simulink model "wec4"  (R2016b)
settings: Solver=ode4  StartTime=0  StopTime=1000  FixedStep=0.005  MaxStep=0.005  RelTol=1e-3  EnableMultiTasking=on
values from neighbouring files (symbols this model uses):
  arAdaptiveLawData = 1/2*zModelSimple.zModelPto.arFreq.*     zModelSimple.zModelPto.arMagnitude./     cos(zModelSimple.zModelPto.arPhase*pi/180+pi/2)    [IMPACT_Control.m]
  arAdaptiveLawDataX = 1/2*zModelSimpleX.zModelPto.arFreq.*         zModelSimpleX.zModelPto.arMagnitude./         cos(zModelSimpleX.zModelPto.arPhase*pi/180+pi/2)    [IMPACT_Control.m]
  arControllerRampGain = [0,0,1,1]    [IMPACT_Control.m]
  arControllerRampTime = [0 rStartRampTime rStartRampTime+rRampTimeLength 8000]    [IMPACT_Control.m]
  arEkfInitialisation = zeros(1,11)    [IMPACT_Control.m]
  arEkfInitialisationX = zeros(1,11)    [IMPACT_Control.m]
  arFrequency = zModelSimple.zModelPto.arFreq    [IMPACT_Control.m]
  arFrequencyRange = zModelSimple.zModelPto.arFreq    [IMPACT_Control.m]
  arFrequencyX = zModelSimpleX.zModelPto.arFreq    [IMPACT_Control.m]
  arImpedance = 1./zModelSimple.zModelPto.arMagnitude./zModelSimple.zModelPto.arFreq    [IMPACT_Control.m]
  arImpedanceX = 1./zModelSimpleX.zModelPto.arMagnitude./zModelSimpleX.zModelPto.arFreq    [IMPACT_Control.m]
  CentralPTOPreload = -1.6113e+07    (= -16113000)    [wecSimInputFile.m]
  F1 = [4.243 2.375 -12.243]    [wecSimInputFile.m]
  F2 = [4.243 -2.375 -12.243]    [wecSimInputFile.m]
  F3 = [-4.243 -2.375 -12.243]    [wecSimInputFile.m]
  F4 = [-4.243 2.375 -12.243]    [wecSimInputFile.m]
  FC = [0 0 -14]    [wecSimInputFile.m]
  iAdaptiveDamping = 0    [wec4IMPACT_Project.m]    (also in IMPACT_Control.m = handles.iAdaptiveDamping; wec1_IMPACT_Project.m; wec2_IMPACT_Project.m; wec3_IMPACT_Project.m)
  iControlType = 2    [wec4IMPACT_Project.m]    (also in IMPACT_Control.m = handles.iControlType; wec1_IMPACT_Project.m = 1; wec2_IMPACT_Project.m = 1; wec3_IMPACT_Project.m = 1)
  iPtoPositionConstraint = 1    [wec4IMPACT_Project.m]    (also in IMPACT_Control.m = handles.iPtoPositionConstraint; wec1_IMPACT_Project.m = 0; wec2_IMPACT_Project.m; wec3_IMPACT_Project.m)
  iSensorNoise = 0    [IMPACT_Control.m]
  m = m+1    (= 2)    [checkParamFile.m]
  PTOrotation = atan((T1(2)-F1(2))/(T1(1)-F1(1)))    [wecSimInputFile.m]
  rCogFloater = -8    [wec4_IMPACT_Model.m]    (also in paramInitial.m = get( handles.edit_rCogFloater, 'String' ); wec1_IMPACT_Model.m = -18; wec2_IMPACT_Model.m = -8.5; wec3_IMPACT_Model.m = -0.7)
  rCogSpar = -36.6    [wec4_IMPACT_Model.m]    (also in paramInitial.m = get( handles.edit_rCogSpar, 'String' ); wec3_IMPACT_Model.m = -21.3; wec3_IMPACT_Model2.m = -21.3)
  rDisplacementLimit = 10.000000    (= 10)    [wec4IMPACT_Project.m]    (also in IMPACT_Control.m = getValue(handles.edit_displacementLimit); wec1_IMPACT_Project.m; wec2_IMPACT_Project.m; wec3_IMPACT_Project.m = 3)
  rDisplacementLimitX = 10.000000    (= 10)    [wec4IMPACT_Project.m]    (also in IMPACT_Control.m = getValue(handles.edit_displacementLimitX); wec1_IMPACT_Project.m = 0; wec2_IMPACT_Project.m; wec3_IMPACT_Project.m = 0)
  rGainForAntiWIndUp = tfControllerDiscrete.rGain    [IMPACT_Control.m]
  rGainForAntiWIndUpX = tfControllerXDiscrete.rGain    [IMPACT_Control.m]
  rMaxForcePto = 300000000.000000    (= 300000000)    [wec4IMPACT_Project.m]    (also in IMPACT_Control.m = getValue(handles.edit_maxForcePto); wec1_IMPACT_Project.m = 1e+15; wec2_IMPACT_Project.m = 1e+15; wec3_IMPACT_Project.m = 1000000000)
  rMinForcePto = -300000000.000000    (= -300000000)    [wec4IMPACT_Project.m]    (also in IMPACT_Control.m = getValue(handles.edit_minForcePto); wec1_IMPACT_Project.m = -1e+15; wec2_IMPACT_Project.m = -1e+15; wec3_IMPACT_Project.m = -1000000000)
  rMooringX = 20000    [wec4_IMPACT_Model.m]    (also in paramInitial.m = get( handles.edit_rMooringX, 'String' ); wec3_IMPACT_Model.m = 10000; wec3_IMPACT_Model2.m = 10000)
  rMooringZ = 10000    [wec4_IMPACT_Model.m]    (also in paramInitial.m = get( handles.edit_rMooringZ, 'String' ); wec3_IMPACT_Model.m = 0; wec3_IMPACT_Model2.m = 0)
  rOutputSampleTime = 0.010000    (= 0.01)    [wec4IMPACT_Project.m]    (also in IMPACT_Control.m = getValue(handles.edit_outputSampleTime); wec1_IMPACT_Project.m; wec2_IMPACT_Project.m; wec3_IMPACT_Project.m)
  rPassiveDampingGain = -604830.000000    (= -604830)    [wec4IMPACT_Project.m]    (also in IMPACT_Control.m = getValue(handles.edit_gainPLD); wec1_IMPACT_Project.m = -214018.1537; wec2_IMPACT_Project.m = -1948070; wec3_IMPACT_Project.m = -519390)
  rPassiveDampingGainX = -278660.000000    (= -278660)    [wec4IMPACT_Project.m]    (also in IMPACT_Control.m = getValue(handles.edit_gainPLDX); wec1_IMPACT_Project.m = 0; wec2_IMPACT_Project.m = 0; wec3_IMPACT_Project.m = 0)
  rTetherPretension = 1.6113e+07    (= 16113000)    [wec4_IMPACT_Model.m]    (also in paramInitial.m = get( handles.edit_rTetherPretension, 'String' ); wec3_IMPACT_Model.m = 0; wec3_IMPACT_Model2.m = 0)
  rTetherSpring = 500000    [wec4_IMPACT_Model.m]    (also in paramInitial.m = get( handles.edit_rTetherSpring, 'String' ); wec3_IMPACT_Model.m = 0; wec3_IMPACT_Model2.m = 0)
  rUpperFrequencyLimit = EKFFloater.upperFreq    [IMPACT_Control.m]
  rXf = 4.243    [wec4AdditionalParams.m]
  rXs = 16.075    [wec4AdditionalParams.m]
  rYf = 2.375    [wec4AdditionalParams.m]
  rYs = 16.075    [wec4AdditionalParams.m]
  rZf = 4.243    [wec4AdditionalParams.m]
  rZs = 2.4350    (= 2.435)    [wec4AdditionalParams.m]
  rZTetherF = 6    [wec4AdditionalParams.m]
  rZTetherS = 2.4350    (= 2.435)    [wec4AdditionalParams.m]
  s = tf('s')    [wec4_IMPACT_Model.m]    (also in IMPACT_Control.m; wec1_IMPACT_Model.m; wec2_IMPACT_Model.m; wec3_IMPACT_Model.m)
  SidePTO1Preload = PreloadPTOCorner    (= 0)    [wecSimInputFile.m]
  SidePTO2Preload = PreloadPTOCorner    (= 0)    [wecSimInputFile.m]
  SidePTO3Preload = PreloadPTOCorner    (= 0)    [wecSimInputFile.m]
  SidePTO4Preload = PreloadPTOCorner    (= 0)    [wecSimInputFile.m]
  simu = simulationClass()    [wecSimInputFile.m]
  T1 = [16.075 16.075 -34.165]    [wecSimInputFile.m]
  T2 = [16.075 -16.075 -34.165]    [wecSimInputFile.m]
  T3 = [-16.075 -16.075 -34.165]    [wecSimInputFile.m]
  T4 = [-16.075 16.075 -34.165]    [wecSimInputFile.m]
  TC = [0 0 -34.165]    [wecSimInputFile.m]
  waves = waveClass('irregular')    [wecSimInputFile.m]
  Z = magPhaseToComplex(zModelTf)    [IMPACT_Control.m]
undefined symbols (not defined in the file or in its folder): arControllerDiscreteDen, arControllerDiscreteNum, arControllerDiscreteXDen, arControllerDiscreteXNum, arExcForceFloaterDen, arExcForceFloaterNum, arExcForceFloaterXDen, arExcForceFloaterXNum, arExcForceSparDen, arExcForceSparNum, arExcForceSparXDen, arExcForceSparXNum, arFexcFloaterDen, arFexcFloaterNum, arFexcFloaterXDen, arFexcFloaterXNum, arFexcSparDen, arFexcSparNum, arFexcSparXDen, arFexcSparXNum, Body, body, constraint, CTTime, deg, Elements, geometry, IRKB, kg, lenJ, mooring, N, pto, rAccelerationGainFloater, rAccelerationGainFloaterX, rAccelerationGainSpar, rAccelerationGainSparX, rad, rBuoyancyGainFloater, rBuoyancyGainFloaterX, rBuoyancyGainSpar, rBuoyancyGainSparX, rDampingGainFloater, rDampingGainFloaterX, rDampingGainSpar, rDampingGainSparX, Rigid, rMaxFocePto, wec4_float, wec4_reactor, WECSim_Lib, X, Y
libraries: nesl_utility x380, sm_lib x170, vrlib x91, simulink x12, WECSim_Lib x4
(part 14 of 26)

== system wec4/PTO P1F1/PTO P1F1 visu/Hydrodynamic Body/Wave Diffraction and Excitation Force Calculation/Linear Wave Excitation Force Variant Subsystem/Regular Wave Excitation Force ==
  note: Calculates the wave force, F_wave, for the case of Regular Waves. F_wave = A * cos(w * t) * Re{Fext} - A * sin(w * t) * Im{Fext}
  In1 : Inport
  Add : Sum
  Add1 : Sum  Inputs=+-
  Constant : Constant  Value=pi/2
  Excitation Imaginary Part : Constant  Value=body.hydroForce.fExt.im(1,:)  VectorParams1D=off
  Excitation Real Part : Constant  Value=body.hydroForce.fExt.re(1,:)  VectorParams1D=off
  Product : Product
  Product1 : Product  Inputs=3
  Product2 : Product  Inputs=3
  Sine Wave Function : Sin  TimeSource=Use external signal  SampleTime=0
  Sine Wave Function1 : Sin  TimeSource=Use external signal  SampleTime=0
  Wave Amplitude : Constant  Value=waves.A(1,:)
  Wave Frequency : Constant  Value=waves.w(1,:)
  Out1 : Outport
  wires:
  Constant/1 -> Add/2
  Add/1 -> Sine Wave Function1/1
  Wave Amplitude/1 -> Product1/1, Product2/1  "A"
  Add1/1 -> Out1/1
  Product2/1 -> Add1/2
  Product1/1 -> Add1/1
  Excitation Real Part/1 -> Product1/2  "Re{Fext}"
  Excitation Imaginary Part/1 -> Product2/3  "Im{Fext}"
  Sine Wave Function/1 -> Product2/2  "sin(wt)"
  Sine Wave Function1/1 -> Product1/3  "cos(w*t)"
  Product/1 -> Add/1, Sine Wave Function/1
  Wave Frequency/1 -> Product/2  "w"
  In1/1 -> Product/1  "t"

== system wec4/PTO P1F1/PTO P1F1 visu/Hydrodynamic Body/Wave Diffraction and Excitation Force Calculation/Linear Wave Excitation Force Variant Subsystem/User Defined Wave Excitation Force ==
  note: Calculates the wave force, F_wave, for the case of User Defined Waves. F_wave = convolution calculation [1x6]
  InputWaveForceTimeHistory : FromWorkspace  VariableName=[waves.waveAmpTime(:,1),body.hydroForce.userDefinedFe]  SampleTime=0
  Out1 : Outport
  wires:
  InputWaveForceTimeHistory/1 -> Out1/1

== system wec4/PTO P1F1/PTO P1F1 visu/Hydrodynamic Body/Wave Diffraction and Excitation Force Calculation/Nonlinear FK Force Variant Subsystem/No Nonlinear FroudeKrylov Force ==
  Constant : Constant  Value=[0 0 0 0 0 0]
  Out1 : Outport
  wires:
  Constant/1 -> Out1/1

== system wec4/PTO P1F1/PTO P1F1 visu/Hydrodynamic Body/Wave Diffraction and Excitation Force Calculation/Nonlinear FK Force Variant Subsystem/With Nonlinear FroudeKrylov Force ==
  In1 : Inport
  In2 : Inport  Port=2
  In3 : Inport  Port=3
  Add : Sum  Inputs=+-
  Center of Gravity : Constant  Value=body.hydroData.properties.cg
  Center of Gravity1 : Constant  Value=body.hydroData.properties.cg
  Constant : Constant  Value=[0 0 0]
  Deep Water Flag : Constant  Value=waves.deepWaterWave
  Diffraction and Excitation Forces : MATLAB Function  TreatAsAtomicUnit=on
  Frequency Spacing : Constant  Value=waves.dw
  Gravity : Constant  Value=simu.g
  Mux : Mux  Inputs=2
  STL Areas : Constant  Value=body.bodyGeometry.area
  STL Centers : Constant  Value=body.bodyGeometry.center
  STL Normal Vectors : Constant  Value=body.bodyGeometry.norm
  To Workspace : ToWorkspace  VariableName=body4_wavenonlinearpressure_out  SaveFormat=Structure With Time  SampleTime=-1
  To Workspace1 : ToWorkspace  VariableName=body4_wavelinearpressure_out  SaveFormat=Structure With Time  SampleTime=-1
  Water Density : Constant  Value=simu.rho
  Water Depth : Constant  Value=waves.waterDepth
  Wave Amplitude : Constant  Value=waves.A
  Wave Frequency : Constant  Value=waves.w
  Wave Number : Constant  Value=waves.k
  Wave Random Phase : Constant  Value=waves.phase
  Wave Type Number : Constant  Value=waves.typeNum
  Out1 : Outport
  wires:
  STL Areas/1 -> Diffraction and Excitation Forces/5(area)
  Diffraction and Excitation Forces/2(wp) -> To Workspace/1
  Diffraction and Excitation Forces/3(wpMeanFS) -> To Workspace1/1
  In2/1 -> Add/1
  Constant/1 -> Mux/2
  Center of Gravity/1 -> Mux/1  "cg"
  Mux/1 -> Add/2
  Add/1 -> Diffraction and Excitation Forces/1(x)  "x_cg"
  Deep Water Flag/1 -> Diffraction and Excitation Forces/13(deepWaterWave)
  Wave Random Phase/1 -> Diffraction and Excitation Forces/17(phaseRand)
  Water Depth/1 -> Diffraction and Excitation Forces/12(wDepth)
  Wave Number/1 -> Diffraction and Excitation Forces/14(k)
  Wave Type Number/1 -> Diffraction and Excitation Forces/15(typeNum)
  Frequency Spacing/1 -> Diffraction and Excitation Forces/11(dw)
  Wave Frequency/1 -> Diffraction and Excitation Forces/10(w)
  Wave Amplitude/1 -> Diffraction and Excitation Forces/9(AH)
  In1/1 -> Diffraction and Excitation Forces/16(t)
  In3/1 -> Diffraction and Excitation Forces/2(elv)
  STL Centers/1 -> Diffraction and Excitation Forces/3(center)
  STL Normal Vectors/1 -> Diffraction and Excitation Forces/4(tnorm)
  Water Density/1 -> Diffraction and Excitation Forces/6(rho)
  Gravity/1 -> Diffraction and Excitation Forces/7(g)
  Diffraction and Excitation Forces/1(f) -> Out1/1
  Center of Gravity1/1 -> Diffraction and Excitation Forces/8(cg)

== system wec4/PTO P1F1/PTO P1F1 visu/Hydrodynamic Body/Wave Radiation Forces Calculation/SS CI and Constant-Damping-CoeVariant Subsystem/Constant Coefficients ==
  In1 : Inport
  Product : Product  Multiplication=Matrix(*)
  Radiation Damping Matrix : Constant  Value=body.hydroForce.fDamping
  Out1 : Outport
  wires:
  In1/1 -> Product/2
  Product/1 -> Out1/1  "F_Single Frequency"
  Radiation Damping Matrix/1 -> Product/1

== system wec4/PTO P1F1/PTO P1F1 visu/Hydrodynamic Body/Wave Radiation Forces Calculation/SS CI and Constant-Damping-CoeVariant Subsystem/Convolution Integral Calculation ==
  In1 : Inport
  MATLAB Function : MATLAB Function  TreatAsAtomicUnit=on  SystemSampleTime=simu.CTTime(2) - simu.CTTime(1)
  Rate Transition : RateTransition
  Reshape : Reshape
  Out1 : Outport
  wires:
  Rate Transition/1 -> Reshape/1
  MATLAB Function/1(F_FM) -> Rate Transition/1
  Reshape/1 -> Out1/1
  In1/1 -> MATLAB Function/1(v)

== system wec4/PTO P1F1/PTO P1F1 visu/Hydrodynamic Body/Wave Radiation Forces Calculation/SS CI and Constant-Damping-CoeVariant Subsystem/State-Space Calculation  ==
  In1 : Inport
  State-Space : StateSpace  A=body.hydroForce.ssRadf.A  B=body.hydroForce.ssRadf.B  C=body.hydroForce.ssRadf.C  D=body.hydroForce.ssRadf.D  X0=0
  Out1 : Outport
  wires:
  State-Space/1 -> Out1/1
  In1/1 -> State-Space/1  "x"

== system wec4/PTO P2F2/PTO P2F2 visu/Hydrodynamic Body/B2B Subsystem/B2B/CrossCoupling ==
  note: CrossCoupling block is updated by its mask initialization, which is only called on when a simulation is run. 'From' blocks are automatically created and connected based on the number of bodies in the simulation.
  Mux1 : Mux  Inputs=2
  Mux2 : Mux  Inputs=2
  vel : Outport
  acc : Outport  Port=2
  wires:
  [acc2] -> Mux2/2
  Mux2/1 -> acc/1
  [acc1] -> Mux2/1
  [vel2] -> Mux1/2
  Mux1/1 -> vel/1
  [vel1] -> Mux1/1

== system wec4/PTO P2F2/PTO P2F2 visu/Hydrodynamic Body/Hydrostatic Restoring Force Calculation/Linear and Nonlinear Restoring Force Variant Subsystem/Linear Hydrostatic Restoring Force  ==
  In1 : Inport
  Add1 : Sum  Inputs=+-
  Add2 : Sum  Inputs=+++
  Add3 : Sum  Inputs=+-
  Assignment (Add Net Bouyancy Force to Z-Direction) : Assignment  IndexOptions=Index vector (dialog)  Indices=3  OutputSizes=1
  Assignment (Add Net Bouyancy Force to Z-Direction)1 : Assignment  IndexOptions=Index vector (dialog)  Indices=3  OutputSizes=1
  Assignment (Add Net Bouyancy Force to Z-Direction)2 : Assignment  IndexOptions=Index vector (dialog)  Indices=4:6  OutputSizes=1
  Body Mass : Constant  Value=body.hydroForce.storage.mass
  Center of Gravity : Constant  Value=body.cg
  Center of Gravity1 : Constant  Value=body.cb
  Constant1 : Constant  Value=[0 0 0 0 0 0]
  Constant2 : Constant  Value=[0 0 0]
  Cross Product : vrlib/Utilities/Cross Product
  Gravity : Constant  Value=simu.g
  Linear Restioring Coefficient Matrix : Constant  Value=body.hydroForce.linearHydroRestCoef
  Product : Product
  Product1 : Product  Inputs=3
  Product2 : Product  Multiplication=Matrix(*)
  Volume : Constant  Value=body.dispVol
  Water Density : Constant  Value=simu.rho
  Out1 : Outport
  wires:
  Assignment (Add Net Bouyancy Force to Z-Direction)2/1 -> Add2/3
  Constant1/1 -> Assignment (Add Net Bouyancy Force to Z-Direction)/1, Assignment (Add Net Bouyancy Force to Z-Direction)2/1
  Cross Product/1 -> Assignment (Add Net Bouyancy Force to Z-Direction)2/2
  Assignment (Add Net Bouyancy Force to Z-Direction)1/1 -> Cross Product/1
  Constant2/1 -> Assignment (Add Net Bouyancy Force to Z-Direction)1/1
  Add3/1 -> Cross Product/2
  Center of Gravity/1 -> Add3/2  "cg"
  Center of Gravity1/1 -> Add3/1  "x"
  Linear Restioring Coefficient Matrix/1 -> Product2/1  "K"
  Product2/1 -> Add2/2  "Linear Restoring Force"
  Add1/1 -> Assignment (Add Net Bouyancy Force to Z-Direction)/2
  Product1/1 -> Assignment (Add Net Bouyancy Force to Z-Direction)1/2, Add1/2  "F_Buoyancy"
  Product/1 -> Add1/1  "F_Gravity"
  Water Density/1 -> Product1/1  "rho"
  Gravity/1 -> Product/1, Product1/2  "g"
  Volume/1 -> Product1/3  "Vol"
  Add2/1 -> Out1/1  "F_Restoring"
  Assignment (Add Net Bouyancy Force to Z-Direction)/1 -> Add2/1  "Net Buoyancy Force"
  Body Mass/1 -> Product/2  "m"
  In1/1 -> Product2/2  "x"

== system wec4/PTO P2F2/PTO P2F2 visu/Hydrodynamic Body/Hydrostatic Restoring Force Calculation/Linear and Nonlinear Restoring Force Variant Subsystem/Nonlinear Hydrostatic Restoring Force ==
  In1 : Inport
  In2 : Inport  Port=2
  Body Mass2 : Constant  Value=body.hydroForce.storage.mass
  Center of Gravity : Constant  Value=body.cg
  Gravity2 : Constant  Value=simu.g
  Rate Transition : RateTransition
  Rate Transition1 : RateTransition
  Restoring Forces : MATLAB Function  TreatAsAtomicUnit=on  SystemSampleTime=simu.dtNL
  STL areas : Constant  Value=body.bodyGeometry.area
  STL centers : Constant  Value=body.bodyGeometry.center
  STL normal vectors : Constant  Value=body.bodyGeometry.norm
  To Workspace1 : ToWorkspace  VariableName=body5_hspressure_out  SaveFormat=Structure With Time  SampleTime=-1
  Water Density1 : Constant  Value=simu.rho
  Out1 : Outport
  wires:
  Rate Transition/1 -> Out1/1
  Restoring Forces/1(f) -> Rate Transition/1
  Rate Transition1/1 -> To Workspace1/1
  Restoring Forces/2(p) -> Rate Transition1/1
  Body Mass2/1 -> Restoring Forces/9(mass)
  STL areas/1 -> Restoring Forces/5(area)
  In2/1 -> Restoring Forces/2(elv)
  STL centers/1 -> Restoring Forces/3(center)
  STL normal vectors/1 -> Restoring Forces/4(tnorm)
  Water Density1/1 -> Restoring Forces/6(rho)
  Gravity2/1 -> Restoring Forces/7(g)  "g"
  Center of Gravity/1 -> Restoring Forces/8(cg)
  In1/1 -> Restoring Forces/1(x)

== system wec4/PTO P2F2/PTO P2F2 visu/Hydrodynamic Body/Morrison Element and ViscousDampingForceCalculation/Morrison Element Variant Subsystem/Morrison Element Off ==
  Constant : Constant  Value=[0 0 0 0 0 0]
  morison_force : Outport
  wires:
  Constant/1 -> morison_force/1

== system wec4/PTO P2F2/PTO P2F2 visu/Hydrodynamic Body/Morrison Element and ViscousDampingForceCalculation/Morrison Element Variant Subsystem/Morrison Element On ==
  note: 1) Add Subsystem or Model blocks as valid variant choices. 2) You cannot connect blocks at this level. At simulation, connectivity is automatically determined, based on the active variant and port name matching.
  displacement : Inport
  velocity : Inport  Port=2
  acceleration : Inport  Port=3
  time : Inport  Port=4
  Irregular Wave Morison Force : Subsystem  TreatAsAtomicUnit=on  SystemSampleTime=simu.dtME  VariantControl=sv_irregularWaves
  No Wave Morison Force : Subsystem  VariantControl=sv_noWave
  Regular Wave Morison Force : Subsystem  TreatAsAtomicUnit=on  SystemSampleTime=simu.dtME  VariantControl=sv_regularWaves
  morison_force : Outport

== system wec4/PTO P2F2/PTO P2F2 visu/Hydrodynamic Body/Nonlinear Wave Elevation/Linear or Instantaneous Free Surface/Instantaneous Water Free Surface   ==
  In1 : Inport
  In2 : Inport  Port=2
  Center of Gravity : Constant  Value=body.cg
  Frequency Spacing : Constant  Value=waves.dw
  Instantaneous FS : MATLAB Function  TreatAsAtomicUnit=on
  Ramp Time : Constant  Value=simu.rampTime
  STL Centers : Constant  Value=body.bodyGeometry.center
  Wave Amplitude : Constant  Value=waves.A
  Wave Direction : Constant  Value=waves.waveDir
  Wave Frequency : Constant  Value=waves.w
  Wave Number : Constant  Value=waves.k
  Wave Random Phase : Constant  Value=waves.phase
  Wave Type Number : Constant  Value=waves.typeNum
  Out1 : Outport
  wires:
  Wave Amplitude/1 -> Instantaneous FS/4(AH)
  Wave Direction/1 -> Instantaneous FS/12(waveDir)
  In1/1 -> Instantaneous FS/1(x)
  In2/1 -> Instantaneous FS/9(t)
  Frequency Spacing/1 -> Instantaneous FS/6(dw)
  Wave Random Phase/1 -> Instantaneous FS/11(phaseRand)
  Ramp Time/1 -> Instantaneous FS/10(rampT)
  Wave Type Number/1 -> Instantaneous FS/8(typeNum)
  Wave Frequency/1 -> Instantaneous FS/5(w)
  Wave Number/1 -> Instantaneous FS/7(k)
  Center of Gravity/1 -> Instantaneous FS/3(cg)
  STL Centers/1 -> Instantaneous FS/2(center)
  Instantaneous FS/1(f) -> Out1/1

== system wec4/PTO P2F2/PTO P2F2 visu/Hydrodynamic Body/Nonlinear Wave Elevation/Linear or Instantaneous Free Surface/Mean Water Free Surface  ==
  zero : Constant  Value=0
  Out1 : Outport
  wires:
  zero/1 -> Out1/1

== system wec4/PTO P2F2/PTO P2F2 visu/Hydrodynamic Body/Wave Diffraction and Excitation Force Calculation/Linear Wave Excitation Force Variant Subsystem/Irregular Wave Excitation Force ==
  note: Calculates the wave force, F_wave, for the case of Irregular Waves. F_wave = sum( F_wave(i)) where i = each frequency bin.
  In1 : Inport
  Frequency Spacing Delta Omega : Constant  Value=waves.dw  VectorParams1D=off
  Imaginary Part of Wave Excitation : Constant  Value=body.hydroForce.fExt.im  VectorParams1D=off
  MATLAB Function : MATLAB Function  TreatAsAtomicUnit=on
  Random Phase : Constant  Value=waves.phase  VectorParams1D=off
  Real Part of Wave Excitation : Constant  Value=body.hydroForce.fExt.re  VectorParams1D=off
  Wave Frequency : Constant  Value=waves.w  VectorParams1D=off
  Wave Spectrum : Constant  Value=waves.A  VectorParams1D=off
  Out1 : Outport
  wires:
  Frequency Spacing Delta Omega/1 -> MATLAB Function/6(dw)
  In1/1 -> MATLAB Function/7(time)
  Wave Spectrum/1 -> MATLAB Function/1(A)
  Real Part of Wave Excitation/1 -> MATLAB Function/3(fExtRE)
  Imaginary Part of Wave Excitation/1 -> MATLAB Function/4(fExtIM)
  Wave Frequency/1 -> MATLAB Function/2(w)
  MATLAB Function/1(Fext) -> Out1/1
  Random Phase/1 -> MATLAB Function/5(phaseRand)

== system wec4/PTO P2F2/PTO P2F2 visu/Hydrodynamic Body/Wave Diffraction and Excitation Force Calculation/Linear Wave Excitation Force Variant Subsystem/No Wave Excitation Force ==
  Constant : Constant  Value=[0 0 0 0 0 0]
  Out1 : Outport
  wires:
  Constant/1 -> Out1/1

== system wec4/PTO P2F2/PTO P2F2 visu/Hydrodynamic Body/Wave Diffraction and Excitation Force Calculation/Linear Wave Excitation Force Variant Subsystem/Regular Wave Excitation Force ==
  note: Calculates the wave force, F_wave, for the case of Regular Waves. F_wave = A * cos(w * t) * Re{Fext} - A * sin(w * t) * Im{Fext}
  In1 : Inport
  Add : Sum
  Add1 : Sum  Inputs=+-
  Constant : Constant  Value=pi/2
  Excitation Imaginary Part : Constant  Value=body.hydroForce.fExt.im(1,:)  VectorParams1D=off
  Excitation Real Part : Constant  Value=body.hydroForce.fExt.re(1,:)  VectorParams1D=off
  Product : Product
  Product1 : Product  Inputs=3
  Product2 : Product  Inputs=3
  Sine Wave Function : Sin  TimeSource=Use external signal  SampleTime=0
  Sine Wave Function1 : Sin  TimeSource=Use external signal  SampleTime=0
  Wave Amplitude : Constant  Value=waves.A(1,:)
  Wave Frequency : Constant  Value=waves.w(1,:)
  Out1 : Outport
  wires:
  Constant/1 -> Add/2
  Add/1 -> Sine Wave Function1/1
  Wave Amplitude/1 -> Product1/1, Product2/1  "A"
  Add1/1 -> Out1/1
  Product2/1 -> Add1/2
  Product1/1 -> Add1/1
  Excitation Real Part/1 -> Product1/2  "Re{Fext}"
  Excitation Imaginary Part/1 -> Product2/3  "Im{Fext}"
  Sine Wave Function/1 -> Product2/2  "sin(wt)"
  Sine Wave Function1/1 -> Product1/3  "cos(w*t)"
  Product/1 -> Add/1, Sine Wave Function/1
  Wave Frequency/1 -> Product/2  "w"
  In1/1 -> Product/1  "t"

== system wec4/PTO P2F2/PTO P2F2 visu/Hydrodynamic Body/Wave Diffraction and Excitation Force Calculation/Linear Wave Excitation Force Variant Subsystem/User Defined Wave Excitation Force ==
  note: Calculates the wave force, F_wave, for the case of User Defined Waves. F_wave = convolution calculation [1x6]
  InputWaveForceTimeHistory : FromWorkspace  VariableName=[waves.waveAmpTime(:,1),body.hydroForce.userDefinedFe]  SampleTime=0
  Out1 : Outport
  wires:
  InputWaveForceTimeHistory/1 -> Out1/1

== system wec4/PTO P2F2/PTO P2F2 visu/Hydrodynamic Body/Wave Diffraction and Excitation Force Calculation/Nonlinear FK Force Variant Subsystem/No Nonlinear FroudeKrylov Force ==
  Constant : Constant  Value=[0 0 0 0 0 0]
  Out1 : Outport
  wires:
  Constant/1 -> Out1/1

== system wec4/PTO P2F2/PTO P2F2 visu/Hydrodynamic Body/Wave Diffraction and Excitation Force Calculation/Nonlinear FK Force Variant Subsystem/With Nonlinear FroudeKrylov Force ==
  In1 : Inport
  In2 : Inport  Port=2
  In3 : Inport  Port=3
  Add : Sum  Inputs=+-
  Center of Gravity : Constant  Value=body.hydroData.properties.cg
  Center of Gravity1 : Constant  Value=body.hydroData.properties.cg
  Constant : Constant  Value=[0 0 0]
  Deep Water Flag : Constant  Value=waves.deepWaterWave
  Diffraction and Excitation Forces : MATLAB Function  TreatAsAtomicUnit=on
  Frequency Spacing : Constant  Value=waves.dw
  Gravity : Constant  Value=simu.g
  Mux : Mux  Inputs=2
  STL Areas : Constant  Value=body.bodyGeometry.area
  STL Centers : Constant  Value=body.bodyGeometry.center
  STL Normal Vectors : Constant  Value=body.bodyGeometry.norm
  To Workspace : ToWorkspace  VariableName=body5_wavenonlinearpressure_out  SaveFormat=Structure With Time  SampleTime=-1
  To Workspace1 : ToWorkspace  VariableName=body5_wavelinearpressure_out  SaveFormat=Structure With Time  SampleTime=-1
  Water Density : Constant  Value=simu.rho
  Water Depth : Constant  Value=waves.waterDepth
  Wave Amplitude : Constant  Value=waves.A
  Wave Frequency : Constant  Value=waves.w
  Wave Number : Constant  Value=waves.k
  Wave Random Phase : Constant  Value=waves.phase
  Wave Type Number : Constant  Value=waves.typeNum
  Out1 : Outport
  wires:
  STL Areas/1 -> Diffraction and Excitation Forces/5(area)
  Diffraction and Excitation Forces/2(wp) -> To Workspace/1
  Diffraction and Excitation Forces/3(wpMeanFS) -> To Workspace1/1
  In2/1 -> Add/1
  Constant/1 -> Mux/2
  Center of Gravity/1 -> Mux/1  "cg"
  Mux/1 -> Add/2
  Add/1 -> Diffraction and Excitation Forces/1(x)  "x_cg"
  Deep Water Flag/1 -> Diffraction and Excitation Forces/13(deepWaterWave)
  Wave Random Phase/1 -> Diffraction and Excitation Forces/17(phaseRand)
  Water Depth/1 -> Diffraction and Excitation Forces/12(wDepth)
  Wave Number/1 -> Diffraction and Excitation Forces/14(k)
  Wave Type Number/1 -> Diffraction and Excitation Forces/15(typeNum)
  Frequency Spacing/1 -> Diffraction and Excitation Forces/11(dw)
  Wave Frequency/1 -> Diffraction and Excitation Forces/10(w)
  Wave Amplitude/1 -> Diffraction and Excitation Forces/9(AH)
  In1/1 -> Diffraction and Excitation Forces/16(t)
  In3/1 -> Diffraction and Excitation Forces/2(elv)
  STL Centers/1 -> Diffraction and Excitation Forces/3(center)
  STL Normal Vectors/1 -> Diffraction and Excitation Forces/4(tnorm)
  Water Density/1 -> Diffraction and Excitation Forces/6(rho)
  Gravity/1 -> Diffraction and Excitation Forces/7(g)
  Diffraction and Excitation Forces/1(f) -> Out1/1
  Center of Gravity1/1 -> Diffraction and Excitation Forces/8(cg)

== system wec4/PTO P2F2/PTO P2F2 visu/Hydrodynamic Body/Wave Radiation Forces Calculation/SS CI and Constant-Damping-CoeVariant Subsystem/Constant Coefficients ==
  In1 : Inport
  Product : Product  Multiplication=Matrix(*)
  Radiation Damping Matrix : Constant  Value=body.hydroForce.fDamping
  Out1 : Outport
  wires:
  In1/1 -> Product/2
  Product/1 -> Out1/1  "F_Single Frequency"
  Radiation Damping Matrix/1 -> Product/1

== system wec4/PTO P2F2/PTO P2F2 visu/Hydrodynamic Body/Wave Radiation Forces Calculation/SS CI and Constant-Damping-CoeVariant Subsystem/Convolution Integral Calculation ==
  In1 : Inport
  MATLAB Function : MATLAB Function  TreatAsAtomicUnit=on  SystemSampleTime=simu.CTTime(2) - simu.CTTime(1)
  Rate Transition : RateTransition
  Reshape : Reshape
  Out1 : Outport
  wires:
  Rate Transition/1 -> Reshape/1
  MATLAB Function/1(F_FM) -> Rate Transition/1
  Reshape/1 -> Out1/1
  In1/1 -> MATLAB Function/1(v)

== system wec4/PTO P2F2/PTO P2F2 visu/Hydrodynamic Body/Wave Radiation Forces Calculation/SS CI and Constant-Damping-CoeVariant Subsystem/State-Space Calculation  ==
  In1 : Inport
  State-Space : StateSpace  A=body.hydroForce.ssRadf.A  B=body.hydroForce.ssRadf.B  C=body.hydroForce.ssRadf.C  D=body.hydroForce.ssRadf.D  X0=0
  Out1 : Outport
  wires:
  State-Space/1 -> Out1/1
  In1/1 -> State-Space/1  "x"

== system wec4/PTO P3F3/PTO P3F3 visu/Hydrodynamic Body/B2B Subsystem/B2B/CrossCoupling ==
  note: CrossCoupling block is updated by its mask initialization, which is only called on when a simulation is run. 'From' blocks are automatically created and connected based on the number of bodies in the simulation.
  Mux1 : Mux  Inputs=2
  Mux2 : Mux  Inputs=2
  vel : Outport
  acc : Outport  Port=2
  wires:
  [acc2] -> Mux2/2
  Mux2/1 -> acc/1
  [acc1] -> Mux2/1
  [vel2] -> Mux1/2
  Mux1/1 -> vel/1
  [vel1] -> Mux1/1

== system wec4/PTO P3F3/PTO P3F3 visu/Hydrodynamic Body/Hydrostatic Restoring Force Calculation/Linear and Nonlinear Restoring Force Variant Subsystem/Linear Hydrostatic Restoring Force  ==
  In1 : Inport
  Add1 : Sum  Inputs=+-
  Add2 : Sum  Inputs=+++
  Add3 : Sum  Inputs=+-
  Assignment (Add Net Bouyancy Force to Z-Direction) : Assignment  IndexOptions=Index vector (dialog)  Indices=3  OutputSizes=1
  Assignment (Add Net Bouyancy Force to Z-Direction)1 : Assignment  IndexOptions=Index vector (dialog)  Indices=3  OutputSizes=1
  Assignment (Add Net Bouyancy Force to Z-Direction)2 : Assignment  IndexOptions=Index vector (dialog)  Indices=4:6  OutputSizes=1
  Body Mass : Constant  Value=body.hydroForce.storage.mass
  Center of Gravity : Constant  Value=body.cg
  Center of Gravity1 : Constant  Value=body.cb
  Constant1 : Constant  Value=[0 0 0 0 0 0]
  Constant2 : Constant  Value=[0 0 0]
  Cross Product : vrlib/Utilities/Cross Product
  Gravity : Constant  Value=simu.g
  Linear Restioring Coefficient Matrix : Constant  Value=body.hydroForce.linearHydroRestCoef
  Product : Product
  Product1 : Product  Inputs=3
  Product2 : Product  Multiplication=Matrix(*)
  Volume : Constant  Value=body.dispVol
  Water Density : Constant  Value=simu.rho
  Out1 : Outport
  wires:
  Assignment (Add Net Bouyancy Force to Z-Direction)2/1 -> Add2/3
  Constant1/1 -> Assignment (Add Net Bouyancy Force to Z-Direction)/1, Assignment (Add Net Bouyancy Force to Z-Direction)2/1
  Cross Product/1 -> Assignment (Add Net Bouyancy Force to Z-Direction)2/2
  Assignment (Add Net Bouyancy Force to Z-Direction)1/1 -> Cross Product/1
  Constant2/1 -> Assignment (Add Net Bouyancy Force to Z-Direction)1/1
  Add3/1 -> Cross Product/2
  Center of Gravity/1 -> Add3/2  "cg"
  Center of Gravity1/1 -> Add3/1  "x"
  Linear Restioring Coefficient Matrix/1 -> Product2/1  "K"
  Product2/1 -> Add2/2  "Linear Restoring Force"
  Add1/1 -> Assignment (Add Net Bouyancy Force to Z-Direction)/2
  Product1/1 -> Assignment (Add Net Bouyancy Force to Z-Direction)1/2, Add1/2  "F_Buoyancy"
  Product/1 -> Add1/1  "F_Gravity"
  Water Density/1 -> Product1/1  "rho"
  Gravity/1 -> Product/1, Product1/2  "g"
  Volume/1 -> Product1/3  "Vol"
  Add2/1 -> Out1/1  "F_Restoring"
  Assignment (Add Net Bouyancy Force to Z-Direction)/1 -> Add2/1  "Net Buoyancy Force"
  Body Mass/1 -> Product/2  "m"
  In1/1 -> Product2/2  "x"

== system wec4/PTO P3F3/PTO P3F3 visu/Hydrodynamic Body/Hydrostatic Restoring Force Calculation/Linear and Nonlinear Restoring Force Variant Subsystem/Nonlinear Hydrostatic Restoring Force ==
  In1 : Inport
  In2 : Inport  Port=2
  Body Mass2 : Constant  Value=body.hydroForce.storage.mass
  Center of Gravity : Constant  Value=body.cg
  Gravity2 : Constant  Value=simu.g
  Rate Transition : RateTransition
  Rate Transition1 : RateTransition
  Restoring Forces : MATLAB Function  TreatAsAtomicUnit=on  SystemSampleTime=simu.dtNL
  STL areas : Constant  Value=body.bodyGeometry.area
  STL centers : Constant  Value=body.bodyGeometry.center
  STL normal vectors : Constant  Value=body.bodyGeometry.norm
  To Workspace1 : ToWorkspace  VariableName=body6_hspressure_out  SaveFormat=Structure With Time  SampleTime=-1
  Water Density1 : Constant  Value=simu.rho
  Out1 : Outport
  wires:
  Rate Transition/1 -> Out1/1
  Restoring Forces/1(f) -> Rate Transition/1
  Rate Transition1/1 -> To Workspace1/1
  Restoring Forces/2(p) -> Rate Transition1/1
  Body Mass2/1 -> Restoring Forces/9(mass)
  STL areas/1 -> Restoring Forces/5(area)
  In2/1 -> Restoring Forces/2(elv)
  STL centers/1 -> Restoring Forces/3(center)
  STL normal vectors/1 -> Restoring Forces/4(tnorm)
  Water Density1/1 -> Restoring Forces/6(rho)
  Gravity2/1 -> Restoring Forces/7(g)  "g"
  Center of Gravity/1 -> Restoring Forces/8(cg)
  In1/1 -> Restoring Forces/1(x)

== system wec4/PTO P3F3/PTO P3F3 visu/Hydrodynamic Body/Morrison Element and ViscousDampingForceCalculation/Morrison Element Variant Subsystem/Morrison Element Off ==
  Constant : Constant  Value=[0 0 0 0 0 0]
  morison_force : Outport
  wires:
  Constant/1 -> morison_force/1

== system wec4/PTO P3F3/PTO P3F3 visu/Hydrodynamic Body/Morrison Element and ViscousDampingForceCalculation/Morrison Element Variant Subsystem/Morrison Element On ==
  note: 1) Add Subsystem or Model blocks as valid variant choices. 2) You cannot connect blocks at this level. At simulation, connectivity is automatically determined, based on the active variant and port name matching.
  displacement : Inport
  velocity : Inport  Port=2
  acceleration : Inport  Port=3
  time : Inport  Port=4
  Irregular Wave Morison Force : Subsystem  TreatAsAtomicUnit=on  SystemSampleTime=simu.dtME  VariantControl=sv_irregularWaves
  No Wave Morison Force : Subsystem  VariantControl=sv_noWave
  Regular Wave Morison Force : Subsystem  TreatAsAtomicUnit=on  SystemSampleTime=simu.dtME  VariantControl=sv_regularWaves
  morison_force : Outport

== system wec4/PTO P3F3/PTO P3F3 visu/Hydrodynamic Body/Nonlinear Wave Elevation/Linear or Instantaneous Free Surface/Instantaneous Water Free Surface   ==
  In1 : Inport
  In2 : Inport  Port=2
  Center of Gravity : Constant  Value=body.cg
  Frequency Spacing : Constant  Value=waves.dw
  Instantaneous FS : MATLAB Function  TreatAsAtomicUnit=on
  Ramp Time : Constant  Value=simu.rampTime
  STL Centers : Constant  Value=body.bodyGeometry.center
  Wave Amplitude : Constant  Value=waves.A
  Wave Direction : Constant  Value=waves.waveDir
  Wave Frequency : Constant  Value=waves.w
  Wave Number : Constant  Value=waves.k
  Wave Random Phase : Constant  Value=waves.phase
  Wave Type Number : Constant  Value=waves.typeNum
  Out1 : Outport
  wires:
  Wave Amplitude/1 -> Instantaneous FS/4(AH)
  Wave Direction/1 -> Instantaneous FS/12(waveDir)
  In1/1 -> Instantaneous FS/1(x)
  In2/1 -> Instantaneous FS/9(t)
  Frequency Spacing/1 -> Instantaneous FS/6(dw)
  Wave Random Phase/1 -> Instantaneous FS/11(phaseRand)
  Ramp Time/1 -> Instantaneous FS/10(rampT)
  Wave Type Number/1 -> Instantaneous FS/8(typeNum)
  Wave Frequency/1 -> Instantaneous FS/5(w)
  Wave Number/1 -> Instantaneous FS/7(k)
  Center of Gravity/1 -> Instantaneous FS/3(cg)
  STL Centers/1 -> Instantaneous FS/2(center)
  Instantaneous FS/1(f) -> Out1/1

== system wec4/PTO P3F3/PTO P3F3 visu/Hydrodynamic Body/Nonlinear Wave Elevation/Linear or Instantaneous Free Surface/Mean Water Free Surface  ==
  zero : Constant  Value=0
  Out1 : Outport
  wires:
  zero/1 -> Out1/1

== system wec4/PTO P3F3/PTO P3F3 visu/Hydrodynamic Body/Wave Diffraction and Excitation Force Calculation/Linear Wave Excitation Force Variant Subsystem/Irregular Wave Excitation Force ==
  note: Calculates the wave force, F_wave, for the case of Irregular Waves. F_wave = sum( F_wave(i)) where i = each frequency bin.
  In1 : Inport
  Frequency Spacing Delta Omega : Constant  Value=waves.dw  VectorParams1D=off
  Imaginary Part of Wave Excitation : Constant  Value=body.hydroForce.fExt.im  VectorParams1D=off
  MATLAB Function : MATLAB Function  TreatAsAtomicUnit=on
  Random Phase : Constant  Value=waves.phase  VectorParams1D=off
  Real Part of Wave Excitation : Constant  Value=body.hydroForce.fExt.re  VectorParams1D=off
  Wave Frequency : Constant  Value=waves.w  VectorParams1D=off
  Wave Spectrum : Constant  Value=waves.A  VectorParams1D=off
  Out1 : Outport
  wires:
  Frequency Spacing Delta Omega/1 -> MATLAB Function/6(dw)
  In1/1 -> MATLAB Function/7(time)
  Wave Spectrum/1 -> MATLAB Function/1(A)
  Real Part of Wave Excitation/1 -> MATLAB Function/3(fExtRE)
  Imaginary Part of Wave Excitation/1 -> MATLAB Function/4(fExtIM)
  Wave Frequency/1 -> MATLAB Function/2(w)
  MATLAB Function/1(Fext) -> Out1/1
  Random Phase/1 -> MATLAB Function/5(phaseRand)

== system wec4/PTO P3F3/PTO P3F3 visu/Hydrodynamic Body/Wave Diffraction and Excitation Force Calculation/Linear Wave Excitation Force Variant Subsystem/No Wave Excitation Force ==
  Constant : Constant  Value=[0 0 0 0 0 0]
  Out1 : Outport
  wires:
  Constant/1 -> Out1/1

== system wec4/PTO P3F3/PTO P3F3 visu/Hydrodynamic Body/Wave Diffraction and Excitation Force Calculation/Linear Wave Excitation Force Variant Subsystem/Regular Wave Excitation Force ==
  note: Calculates the wave force, F_wave, for the case of Regular Waves. F_wave = A * cos(w * t) * Re{Fext} - A * sin(w * t) * Im{Fext}
  In1 : Inport
  Add : Sum
  Add1 : Sum  Inputs=+-
  Constant : Constant  Value=pi/2
  Excitation Imaginary Part : Constant  Value=body.hydroForce.fExt.im(1,:)  VectorParams1D=off
  Excitation Real Part : Constant  Value=body.hydroForce.fExt.re(1,:)  VectorParams1D=off
  Product : Product
  Product1 : Product  Inputs=3
  Product2 : Product  Inputs=3
  Sine Wave Function : Sin  TimeSource=Use external signal  SampleTime=0
  Sine Wave Function1 : Sin  TimeSource=Use external signal  SampleTime=0
  Wave Amplitude : Constant  Value=waves.A(1,:)
  Wave Frequency : Constant  Value=waves.w(1,:)
  Out1 : Outport
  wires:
  Constant/1 -> Add/2
  Add/1 -> Sine Wave Function1/1
  Wave Amplitude/1 -> Product1/1, Product2/1  "A"
  Add1/1 -> Out1/1
  Product2/1 -> Add1/2
  Product1/1 -> Add1/1
  Excitation Real Part/1 -> Product1/2  "Re{Fext}"
  Excitation Imaginary Part/1 -> Product2/3  "Im{Fext}"
  Sine Wave Function/1 -> Product2/2  "sin(wt)"
  Sine Wave Function1/1 -> Product1/3  "cos(w*t)"
  Product/1 -> Add/1, Sine Wave Function/1
  Wave Frequency/1 -> Product/2  "w"
  In1/1 -> Product/1  "t"

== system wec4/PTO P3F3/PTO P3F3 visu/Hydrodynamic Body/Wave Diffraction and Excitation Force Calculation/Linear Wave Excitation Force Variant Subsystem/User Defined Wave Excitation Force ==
  note: Calculates the wave force, F_wave, for the case of User Defined Waves. F_wave = convolution calculation [1x6]
  InputWaveForceTimeHistory : FromWorkspace  VariableName=[waves.waveAmpTime(:,1),body.hydroForce.userDefinedFe]  SampleTime=0
  Out1 : Outport
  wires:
  InputWaveForceTimeHistory/1 -> Out1/1

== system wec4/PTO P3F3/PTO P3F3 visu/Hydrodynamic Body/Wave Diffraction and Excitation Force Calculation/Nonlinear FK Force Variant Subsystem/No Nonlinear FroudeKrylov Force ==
  Constant : Constant  Value=[0 0 0 0 0 0]
  Out1 : Outport
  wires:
  Constant/1 -> Out1/1

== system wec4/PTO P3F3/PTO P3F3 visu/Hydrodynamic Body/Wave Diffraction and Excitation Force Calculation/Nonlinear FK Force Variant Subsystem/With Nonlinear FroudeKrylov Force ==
  In1 : Inport
  In2 : Inport  Port=2
  In3 : Inport  Port=3
  Add : Sum  Inputs=+-
  Center of Gravity : Constant  Value=body.hydroData.properties.cg
  Center of Gravity1 : Constant  Value=body.hydroData.properties.cg
  Constant : Constant  Value=[0 0 0]
  Deep Water Flag : Constant  Value=waves.deepWaterWave
  Diffraction and Excitation Forces : MATLAB Function  TreatAsAtomicUnit=on
  Frequency Spacing : Constant  Value=waves.dw
  Gravity : Constant  Value=simu.g
  Mux : Mux  Inputs=2
  STL Areas : Constant  Value=body.bodyGeometry.area
  STL Centers : Constant  Value=body.bodyGeometry.center
  STL Normal Vectors : Constant  Value=body.bodyGeometry.norm
  To Workspace : ToWorkspace  VariableName=body6_wavenonlinearpressure_out  SaveFormat=Structure With Time  SampleTime=-1
  To Workspace1 : ToWorkspace  VariableName=body6_wavelinearpressure_out  SaveFormat=Structure With Time  SampleTime=-1
  Water Density : Constant  Value=simu.rho
  Water Depth : Constant  Value=waves.waterDepth
  Wave Amplitude : Constant  Value=waves.A
  Wave Frequency : Constant  Value=waves.w
  Wave Number : Constant  Value=waves.k
  Wave Random Phase : Constant  Value=waves.phase
  Wave Type Number : Constant  Value=waves.typeNum
  Out1 : Outport
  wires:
  STL Areas/1 -> Diffraction and Excitation Forces/5(area)
  Diffraction and Excitation Forces/2(wp) -> To Workspace/1
  Diffraction and Excitation Forces/3(wpMeanFS) -> To Workspace1/1
  In2/1 -> Add/1
  Constant/1 -> Mux/2
  Center of Gravity/1 -> Mux/1  "cg"
  Mux/1 -> Add/2
  Add/1 -> Diffraction and Excitation Forces/1(x)  "x_cg"
  Deep Water Flag/1 -> Diffraction and Excitation Forces/13(deepWaterWave)
  Wave Random Phase/1 -> Diffraction and Excitation Forces/17(phaseRand)
  Water Depth/1 -> Diffraction and Excitation Forces/12(wDepth)
  Wave Number/1 -> Diffraction and Excitation Forces/14(k)
  Wave Type Number/1 -> Diffraction and Excitation Forces/15(typeNum)
  Frequency Spacing/1 -> Diffraction and Excitation Forces/11(dw)
  Wave Frequency/1 -> Diffraction and Excitation Forces/10(w)
  Wave Amplitude/1 -> Diffraction and Excitation Forces/9(AH)
  In1/1 -> Diffraction and Excitation Forces/16(t)
  In3/1 -> Diffraction and Excitation Forces/2(elv)
  STL Centers/1 -> Diffraction and Excitation Forces/3(center)
  STL Normal Vectors/1 -> Diffraction and Excitation Forces/4(tnorm)
  Water Density/1 -> Diffraction and Excitation Forces/6(rho)
  Gravity/1 -> Diffraction and Excitation Forces/7(g)
  Diffraction and Excitation Forces/1(f) -> Out1/1
  Center of Gravity1/1 -> Diffraction and Excitation Forces/8(cg)

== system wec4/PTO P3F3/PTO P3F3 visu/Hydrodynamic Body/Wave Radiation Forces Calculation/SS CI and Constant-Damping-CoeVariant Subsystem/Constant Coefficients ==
  In1 : Inport
  Product : Product  Multiplication=Matrix(*)
  Radiation Damping Matrix : Constant  Value=body.hydroForce.fDamping
  Out1 : Outport
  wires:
  In1/1 -> Product/2
  Product/1 -> Out1/1  "F_Single Frequency"
  Radiation Damping Matrix/1 -> Product/1

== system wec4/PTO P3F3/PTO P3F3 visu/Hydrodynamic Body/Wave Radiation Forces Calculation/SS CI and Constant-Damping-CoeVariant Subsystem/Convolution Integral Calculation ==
  In1 : Inport
  MATLAB Function : MATLAB Function  TreatAsAtomicUnit=on  SystemSampleTime=simu.CTTime(2) - simu.CTTime(1)
  Rate Transition : RateTransition
  Reshape : Reshape
  Out1 : Outport
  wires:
  Rate Transition/1 -> Reshape/1
  MATLAB Function/1(F_FM) -> Rate Transition/1
  Reshape/1 -> Out1/1
  In1/1 -> MATLAB Function/1(v)

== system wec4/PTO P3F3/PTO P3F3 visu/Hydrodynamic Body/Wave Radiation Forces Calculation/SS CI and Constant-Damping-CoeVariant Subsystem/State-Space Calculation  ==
  In1 : Inport
  State-Space : StateSpace  A=body.hydroForce.ssRadf.A  B=body.hydroForce.ssRadf.B  C=body.hydroForce.ssRadf.C  D=body.hydroForce.ssRadf.D  X0=0
  Out1 : Outport
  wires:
  State-Space/1 -> Out1/1
  In1/1 -> State-Space/1  "x"

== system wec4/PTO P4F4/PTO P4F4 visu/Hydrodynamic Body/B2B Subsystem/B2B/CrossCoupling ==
  note: CrossCoupling block is updated by its mask initialization, which is only called on when a simulation is run. 'From' blocks are automatically created and connected based on the number of bodies in the simulation.
  Mux1 : Mux  Inputs=2
  Mux2 : Mux  Inputs=2
  vel : Outport
  acc : Outport  Port=2
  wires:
  [acc2] -> Mux2/2
  Mux2/1 -> acc/1
  [acc1] -> Mux2/1
  [vel2] -> Mux1/2
  Mux1/1 -> vel/1
  [vel1] -> Mux1/1

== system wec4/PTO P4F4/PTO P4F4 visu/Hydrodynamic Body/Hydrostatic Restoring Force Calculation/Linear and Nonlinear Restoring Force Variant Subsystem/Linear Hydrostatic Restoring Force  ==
  In1 : Inport
  Add1 : Sum  Inputs=+-
  Add2 : Sum  Inputs=+++
  Add3 : Sum  Inputs=+-
  Assignment (Add Net Bouyancy Force to Z-Direction) : Assignment  IndexOptions=Index vector (dialog)  Indices=3  OutputSizes=1
  Assignment (Add Net Bouyancy Force to Z-Direction)1 : Assignment  IndexOptions=Index vector (dialog)  Indices=3  OutputSizes=1
  Assignment (Add Net Bouyancy Force to Z-Direction)2 : Assignment  IndexOptions=Index vector (dialog)  Indices=4:6  OutputSizes=1
  Body Mass : Constant  Value=body.hydroForce.storage.mass
  Center of Gravity : Constant  Value=body.cg
  Center of Gravity1 : Constant  Value=body.cb
  Constant1 : Constant  Value=[0 0 0 0 0 0]
  Constant2 : Constant  Value=[0 0 0]
  Cross Product : vrlib/Utilities/Cross Product
  Gravity : Constant  Value=simu.g
  Linear Restioring Coefficient Matrix : Constant  Value=body.hydroForce.linearHydroRestCoef
  Product : Product
  Product1 : Product  Inputs=3
  Product2 : Product  Multiplication=Matrix(*)
  Volume : Constant  Value=body.dispVol
  Water Density : Constant  Value=simu.rho
  Out1 : Outport
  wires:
  Assignment (Add Net Bouyancy Force to Z-Direction)2/1 -> Add2/3
  Constant1/1 -> Assignment (Add Net Bouyancy Force to Z-Direction)/1, Assignment (Add Net Bouyancy Force to Z-Direction)2/1
  Cross Product/1 -> Assignment (Add Net Bouyancy Force to Z-Direction)2/2
  Assignment (Add Net Bouyancy Force to Z-Direction)1/1 -> Cross Product/1
  Constant2/1 -> Assignment (Add Net Bouyancy Force to Z-Direction)1/1
  Add3/1 -> Cross Product/2
  Center of Gravity/1 -> Add3/2  "cg"
  Center of Gravity1/1 -> Add3/1  "x"
  Linear Restioring Coefficient Matrix/1 -> Product2/1  "K"
  Product2/1 -> Add2/2  "Linear Restoring Force"
  Add1/1 -> Assignment (Add Net Bouyancy Force to Z-Direction)/2
  Product1/1 -> Assignment (Add Net Bouyancy Force to Z-Direction)1/2, Add1/2  "F_Buoyancy"
  Product/1 -> Add1/1  "F_Gravity"
  Water Density/1 -> Product1/1  "rho"
  Gravity/1 -> Product/1, Product1/2  "g"
  Volume/1 -> Product1/3  "Vol"
  Add2/1 -> Out1/1  "F_Restoring"
  Assignment (Add Net Bouyancy Force to Z-Direction)/1 -> Add2/1  "Net Buoyancy Force"
  Body Mass/1 -> Product/2  "m"
  In1/1 -> Product2/2  "x"

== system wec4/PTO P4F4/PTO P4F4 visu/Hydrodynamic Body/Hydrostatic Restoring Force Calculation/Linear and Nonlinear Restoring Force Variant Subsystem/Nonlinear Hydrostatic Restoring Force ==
  In1 : Inport
  In2 : Inport  Port=2
  Body Mass2 : Constant  Value=body.hydroForce.storage.mass
  Center of Gravity : Constant  Value=body.cg
  Gravity2 : Constant  Value=simu.g
  Rate Transition : RateTransition
  Rate Transition1 : RateTransition
  Restoring Forces : MATLAB Function  TreatAsAtomicUnit=on  SystemSampleTime=simu.dtNL
  STL areas : Constant  Value=body.bodyGeometry.area
  STL centers : Constant  Value=body.bodyGeometry.center
  STL normal vectors : Constant  Value=body.bodyGeometry.norm
  To Workspace1 : ToWorkspace  VariableName=body7_hspressure_out  SaveFormat=Structure With Time  SampleTime=-1
  Water Density1 : Constant  Value=simu.rho
  Out1 : Outport
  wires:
  Rate Transition/1 -> Out1/1
  Restoring Forces/1(f) -> Rate Transition/1
  Rate Transition1/1 -> To Workspace1/1
  Restoring Forces/2(p) -> Rate Transition1/1
  Body Mass2/1 -> Restoring Forces/9(mass)
  STL areas/1 -> Restoring Forces/5(area)
  In2/1 -> Restoring Forces/2(elv)
  STL centers/1 -> Restoring Forces/3(center)
  STL normal vectors/1 -> Restoring Forces/4(tnorm)
  Water Density1/1 -> Restoring Forces/6(rho)
  Gravity2/1 -> Restoring Forces/7(g)  "g"
  Center of Gravity/1 -> Restoring Forces/8(cg)
  In1/1 -> Restoring Forces/1(x)

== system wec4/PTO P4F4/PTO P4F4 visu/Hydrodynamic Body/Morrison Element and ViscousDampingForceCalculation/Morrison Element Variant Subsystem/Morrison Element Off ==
  Constant : Constant  Value=[0 0 0 0 0 0]
  morison_force : Outport
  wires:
  Constant/1 -> morison_force/1

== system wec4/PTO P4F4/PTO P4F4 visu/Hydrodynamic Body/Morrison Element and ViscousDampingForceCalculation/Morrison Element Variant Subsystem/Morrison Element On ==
  note: 1) Add Subsystem or Model blocks as valid variant choices. 2) You cannot connect blocks at this level. At simulation, connectivity is automatically determined, based on the active variant and port name matching.
  displacement : Inport
  velocity : Inport  Port=2
  acceleration : Inport  Port=3
  time : Inport  Port=4
  Irregular Wave Morison Force : Subsystem  TreatAsAtomicUnit=on  SystemSampleTime=simu.dtME  VariantControl=sv_irregularWaves
  No Wave Morison Force : Subsystem  VariantControl=sv_noWave
  Regular Wave Morison Force : Subsystem  TreatAsAtomicUnit=on  SystemSampleTime=simu.dtME  VariantControl=sv_regularWaves
  morison_force : Outport
